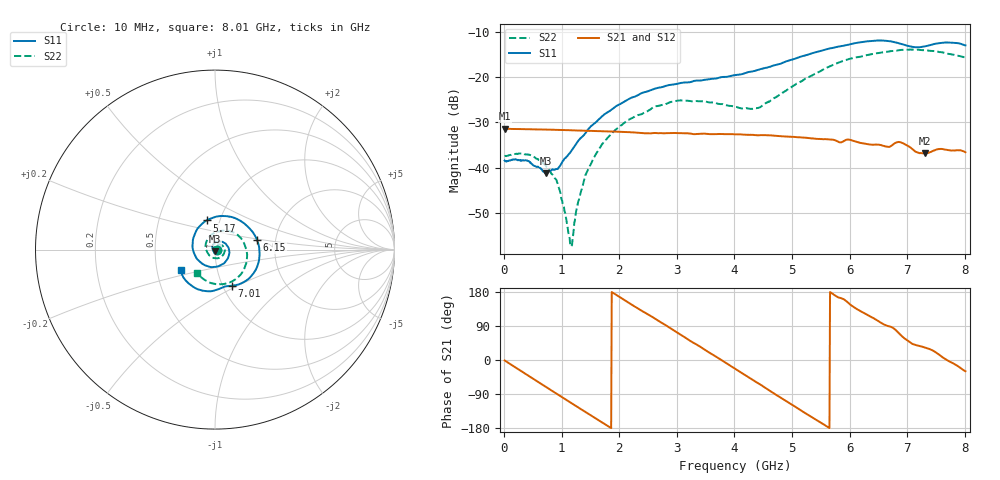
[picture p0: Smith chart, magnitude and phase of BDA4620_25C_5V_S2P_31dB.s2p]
!Agilent Technologies,E5071B,MY42404982,A.09.10
!Date: Wed May 06 09:05:13 2026
!Data & Calibration Information:
!Freq	S11:SOLT2(ON)	S21:SOLT2(ON)	S12:SOLT2(ON)	S22:SOLT2(ON)
# Hz S RI R 50
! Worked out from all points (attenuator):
!   801 points, 10 MHz to 8.01 GHz, reference 50 ohm
!   highest |S21| = -31.37 dB at 10 MHz (marker M1); lowest = -36.8 dB at 7.31 GHz (marker M2)
!   lowest |S11| = -41.2 dB at 720 MHz (marker M3), VSWR 1.02, Z = 49.9 - j0.869 ohm
!   |S11| at or under -10 dB: start of sweep to end of sweep
!   |S22| runs from -57.3 to -13.9 dB; largest |S21 - S12| = 0.00016
!   S11 on the Smith chart (normalised r, x): 10 MHz: 1.02, -0.00; 5.17 GHz: 0.86, +0.29; 6.15 GHz: 1.60, +0.19; 7.01 GHz: 1.10, -0.47; 8.01 GHz: 0.66, -0.16
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1e7  0.012 -0.00071  0.027 -0.000549  0.027 -0.000555  0.0134 -0.000422
4.4e8  0.00828 -0.00825  0.0194 -0.0182  0.0195 -0.0182  0.0131 -0.00471
7.2e8  -0.000854 -0.00871  0.0089 -0.0249  0.00891 -0.0249  0.00835 -0.00671
9.4e8  -0.00883 -0.00441  -0.000711 -0.0261  -0.000737 -0.0262  0.00335 -0.00533
1.16e9  -0.0142 0.00514  -0.0101 -0.0239  -0.0101 -0.0239  -0.00118 -0.000695
1.19e9  -0.0147 0.00672  -0.0112 -0.0233  -0.0113 -0.0234  -0.00162 0.000209
1.35e9  -0.0151 0.0158  -0.0169 -0.0194  -0.0169 -0.0194  -0.00311 0.00494
1.53e9  -0.0112 0.0272  -0.0217 -0.0134  -0.0216 -0.0134  -0.00285 0.0114
1.77e9  0.00127 0.0399  -0.0249 -0.00387  -0.0249 -0.00392  0.0012 0.0204
2.14e9  0.0332 0.0452  -0.0221 0.0111  -0.0222 0.0111  0.0168 0.0287
2.68e9  0.076 0.00812  -0.00565 0.0234  -0.00561 0.0235  0.0443 0.0191
3.08e9  0.0735 -0.0453  0.00998 0.0219  0.0101 0.0219  0.0547 -0.00751
4.01e9  -0.065 -0.0826  0.0215 -0.00919  0.0216 -0.00918  -0.0104 -0.0462
4.43e9  -0.121 -0.00864  0.0104 -0.0203  0.0104 -0.0204  -0.0447 -0.0113
5.17e9  -0.0471 0.1627  -0.0151 -0.0154  -0.0152 -0.0155  -0.00813 0.09
5.35e9  0.00613 0.1836  -0.0186 -0.0101  -0.0185 -0.0101  0.0232 0.1018
6.15e9  0.2339 0.0549  -0.0129 0.0141  -0.0129 0.0141  0.1633 0.0312
6.68e9  0.1959 -0.1548  0.000273 0.017  0.000278 0.017  0.1693 -0.0897
7.01e9  0.0924 -0.2011  0.0111 0.0135  0.0111 0.0136  0.1219 -0.1593
7.31e9  0.0293 -0.2167  0.0121 0.00774  0.0122 0.00778  0.0511 -0.1913
7.65e9  -0.0886 -0.2237  0.0159 0.00101  0.0159 0.000952  -0.0324 -0.1821
8.01e9  -0.1911 -0.1163  0.0129 -0.00736  0.013 -0.00736  -0.1025 -0.1282
